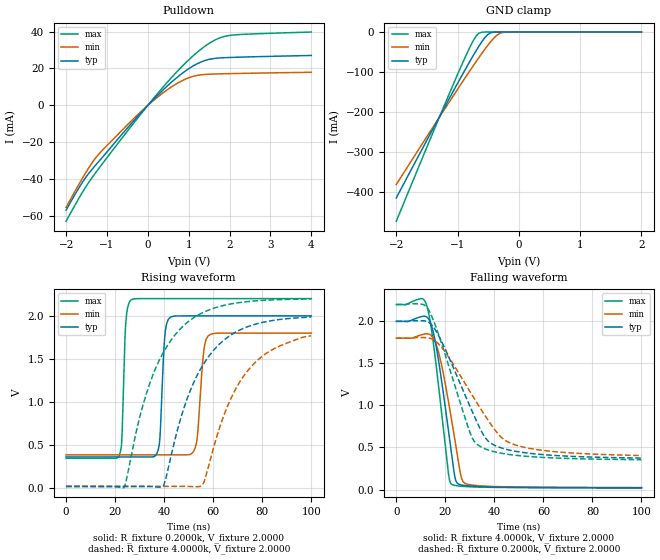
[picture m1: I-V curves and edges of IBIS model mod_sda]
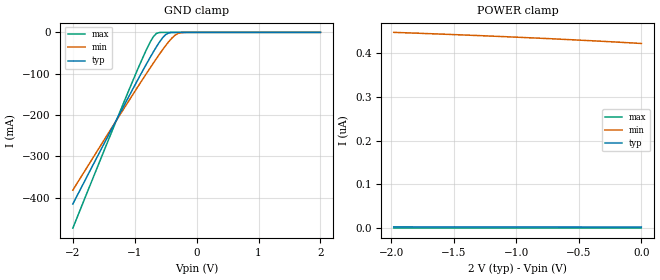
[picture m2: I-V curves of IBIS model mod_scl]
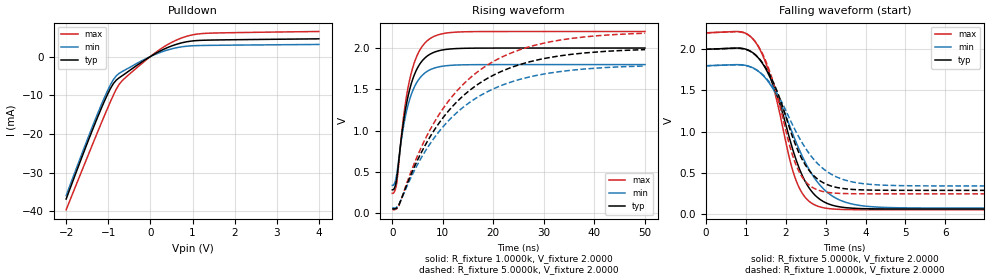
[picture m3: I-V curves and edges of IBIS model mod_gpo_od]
| IBIS (I/O, Buffer, Information, Specification) Model, officially
| electronic behavioral standard for Buffer structures of digital pins.
[IBIS ver]  4.0
[File name] st25dv04kc_so8_2v0.ibs
[File Rev]  1.0
[Date]   5 March 2024
[Notes]
   (Note1)  This IBIS model includes the SO8 package data
   (Note2)  This IBIS model has some Notes about the non-monotonicity
   of the I-V curves, but they are not indicative of problems
   inside the model;
[Disclaimer]
   Customers are solely responsible for all aspects of their
   own product designs or applications using this IBIS Model.
   STMicroelectronics assumes no liability for Custmer Designs
   and applications associated to this IBIS Model.
   In the use of this IBIS Model Customer shall not modify,
   disassemble, alter this Model in whole or in part.
   If Customers do not accept these terms, the IBIS Model
   may not be used. For any problems or modifications please
   contact STMicroelectronics (www.st.com).
[Copyright] (c) 2024 STMicroelectronics
|   Component ST25DV04K
[Component] ST25DV04K
[Manufacturer] STMicroelectronics
[Package]
| variable  typ   min   max
R_pkg   0.0   0.0   0.0
L_pkg   0.0H   0.0H   0.0H
C_pkg   0.0F   0.0F   0.0F
[Pin]  signal_name  model_name   R_pin   L_pin   C_pin
1   VEH   NC   0.0   0.0   0.0
2   AC0   NC   0.0   0.0   0.0
3   AC1   NC   0.0   0.0   0.0
4   VSS   GND   130.95m   2.182nH   0.287pF
5   SDA   mod_sda   130.79m   2.182nH   0.286pF
6   SCL   mod_scl   85.32m   1.589nH   0.354pF
7   GPO   mod_gpo_od   84.54m   1.583nH   0.355pF
8   VCC   POWER   124.14m   2.142nH   0.284pF
| Models and submodels in the file (3): mod_sda (I/O_open_drain), mod_scl (Input), mod_gpo_od (Open_drain)
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|   Model mod_sda
[Model]   mod_sda
Model_type I/O_open_drain
Polarity   Non-Inverting
Enable   Active-Low
Vinl   =   0.500V
Vinh   =   1.500V
Vmeas  =   1.000V
Cref   =   30.0pF
Rref   =   4.0k
Vref   =   2.000V
C_comp   3.063pF   2.925pF   3.207pF
[Model Spec]
Vmeas   1.000V   0.900V   1.100V
Vinl   0.500V   0.450V   0.550V
Vinh   1.500V   1.350V   1.650V
[Temperature Range]  25.0000   85.0000   -40.0000
[Voltage Range]   2.0000V   1.8000V   2.2000V
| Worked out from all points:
|   slope of the pulldown table from 0 to 0.3 V, typ, clamps not added: 44 ohm
|   GND clamp passes 1 mA (typ) near -0.44 V on its own axis
|   rising waveform, R_fixture 0.2000k, V_fixture 2.0000: 20-80 % time 1.54ns typ, 2.1ns min, 1.21ns max; typ from 0.364 V to 2 V
|   rising waveform, R_fixture 4.0000k, V_fixture 2.0000: 20-80 % time 16.8ns typ, 16.6ns min, 16.9ns max; typ from 0.021 V to 1.99 V
|   falling waveform, R_fixture 4.0000k, V_fixture 2.0000: 20-80 % time 5.73ns typ, 6.35ns min, 5.23ns max; typ from 2 V to 0.022 V
|   falling waveform, R_fixture 0.2000k, V_fixture 2.0000: 20-80 % time 14.7ns typ, 18.3ns min, 12.1ns max; typ from 2 V to 0.374 V
[Pulldown]
|Voltage   I(typ)   I(min)   I(max)
-2V       -56.79mA   -55.22mA   -62.78mA
-1.58V    -40.98mA   -38.72mA   -46.34mA
-1.3V     -32.95mA   -29.14mA   -37.16mA
-1.09V    -27.58mA   -23.79mA   -30.96mA
-390mV    -9.491mA   -8.101mA   -10.85mA
170mV     3.93mA     3.244mA    4.596mA
590mV     12.8mA     10.2mA     15.32mA
940mV     18.95mA    14.41mA    23.37mA
1.29V     23.41mA    16.53mA    30.26mA
1.64V     25.46mA    17.02mA    35.37mA
1.99V     25.95mA    17.21mA    37.85mA
4V        27.04mA    17.94mA    39.74mA
[GND_clamp]
|Voltage   I(typ)   I(min)   I(max)
-2V       -415.4mA   -381.8mA   -473.8mA
-1.35V    -227.6mA   -225.9mA   -232.7mA
-950mV    -114.5mA   -131.6mA   -88.58mA
-750mV    -60.32mA   -85.72mA   -23.2mA
-700mV    -47.4mA    -74.51mA   -10.46mA
-650mV    -34.97mA   -63.45mA   -2.549mA
-550mV    -13.06mA   -42.04mA   -27.64uA
-500mV    -5.297mA   -31.88mA   -2.458uA
-450mV    -1.324mA   -22.35mA   -217.9nA
-350mV    -35.28uA   -6.896mA   -1.714nA
-250mV    -802.3nA   -654.1uA   -15.76pA
2V        2.514nA    426.1nA    6.718pA
[Ramp]
| variable   typ   min   max
dV/dt_r   0.5972/2.3539n   0.4569/2.8918n   0.7297/1.3653n
dV/dt_f   0.5671/31.8553n   0.4108/32.1388n   0.7057/23.5150n
R_load = 50.0000
[Rising Waveform]
R_fixture= 0.2000k
V_fixture= 2.0000
V_fixture_min= 1.8000
V_fixture_max= 2.2000
|time   V(typ)   V(min)   V(max)
0s        363.6mV    387.8mV    348mV
21.66ns   363.6mV    387.8mV    378mV
24.4ns    363.6mV    387.8mV    1.937V
26.88ns   363.6mV    387.8mV    2.191V
37.52ns   440.7mV    387.8mV    2.2V
40.24ns   1.757V     387.8mV    2.2V
42.56ns   1.984V     387.8mV    2.2V
52.62ns   2V         466.6mV    2.2V
57.92ns   2V         1.768V     2.2V
100ns     2V         1.8V       2.2V
[Rising Waveform]
R_fixture= 4.0000k
V_fixture= 2.0000
V_fixture_min= 1.8000
V_fixture_max= 2.2000
|time   V(typ)   V(min)   V(max)
0s        21.01mV    22.65mV    19.91mV
23.68ns   21.01mV    22.65mV    8.087mV
31.38ns   21.01mV    22.65mV    967.1mV
39.22ns   15.66mV    22.65mV    1.552V
48.06ns   930.9mV    22.68mV    1.89V
55.46ns   1.415V     31.43mV    2.034V
65.36ns   1.741V     919.7mV    2.128V
73.16ns   1.865V     1.331V     2.163V
83.56ns   1.943V     1.599V     2.185V
100ns     1.986V     1.768V     2.196V
[Falling Waveform]
R_fixture= 4.0000k
V_fixture= 2.0000
V_fixture_min= 1.8000
V_fixture_max= 2.2000
|time   V(typ)   V(min)   V(max)
0s        2V         1.8V       2.2V
12.52ns   2.051V     1.852V     2.179V
14.8ns    1.905V     1.814V     1.811V
17.04ns   1.571V     1.653V     1.284V
21.3ns    696.3mV    1.042V     188.4mV
22.58ns   418.3mV    821.4mV    62.67mV
24.5ns    91.09mV    481.9mV    46.23mV
26.74ns   53.4mV     124.7mV    38.57mV
28.66ns   45.46mV    65.78mV    34.65mV
100ns     21.59mV    23.54mV    20.3mV
[Falling Waveform]
R_fixture= 0.2000k
V_fixture= 2.0000
V_fixture_min= 1.8000
V_fixture_max= 2.2000
|time   V(typ)   V(min)   V(max)
0s        2V         1.8V       2.2V
9.72ns    2.008V     1.807V     2.208V
12.78ns   1.995V     1.804V     2.154V
18.68ns   1.749V     1.683V     1.718V
30.24ns   977.1mV    1.156V     664.1mV
34.44ns   708.7mV    958.8mV    508.4mV
37.24ns   581.8mV    833.1mV    472.7mV
42.84ns   494.9mV    620.4mV    431.7mV
49.84ns   448.8mV    519.2mV    403.7mV
100ns     374.2mV    404.2mV    354.8mV
|   Model mod_scl
[Model]   mod_scl
Model_type Input
Vinl   =   0.500V
Vinh   =   1.500V
C_comp   2.118pF   2.024pF   2.219pF
[Model Spec]
Vinl   0.500V   0.450V   0.550V
Vinh   1.500V   1.350V   1.650V
[Temperature Range]  25.0000   85.0000   -40.0000
[Voltage Range]   2.0000V   1.8000V   2.2000V
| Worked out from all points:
|   GND clamp passes 1 mA (typ) near -0.44 V on its own axis
[GND_clamp]
|Voltage   I(typ)   I(min)   I(max)
-2V       -415.4mA   -381.8mA   -473.8mA
-1.35V    -227.6mA   -225.9mA   -232.7mA
-950mV    -114.5mA   -131.6mA   -88.58mA
-750mV    -60.32mA   -85.72mA   -23.2mA
-700mV    -47.4mA    -74.51mA   -10.46mA
-650mV    -34.97mA   -63.45mA   -2.549mA
-550mV    -13.06mA   -42.04mA   -27.64uA
-500mV    -5.297mA   -31.88mA   -2.458uA
-450mV    -1.324mA   -22.35mA   -217.9nA
-350mV    -35.28uA   -6.896mA   -1.714nA
-250mV    -802.3nA   -654.1uA   -15.76pA
2V        2.514nA    426.1nA    6.718pA
[POWER_clamp]
|Voltage   I(typ)   I(min)   I(max)
-1.98V    2.873nA    448.3nA    11.48pA
-1.77V    2.841nA    446.2nA    11.03pA
-1.38V    2.78nA     441.9nA    10.19pA
-1.11V    2.734nA    438.7nA    9.602pA
-870mV    2.691nA    435.6nA    9.079pA
-840mV    2.686nA    435.3nA    9.014pA
-690mV    2.658nA    433.3nA    8.685pA
-360mV    2.592nA    428.6nA    7.961pA
0V        2.514nA    422.9nA    7.164pA
|   Model mod_gpo_od
[Model]   mod_gpo_od
Model_type Open_drain
Polarity   Non-Inverting
Enable   Active-Low
Vmeas  =   1.000V
Cref   =   30.0pF
Rref   =   5.0k
Vref   =   2.00V
C_comp   2.219pF   2.119pF   2.324pF
[Model Spec]
Vmeas   1.000V   0.900V   1.100V
[Temperature Range]  25.0000   85.0000   -40.0000
[Voltage Range]   2.0000V   1.8000V   2.2000V
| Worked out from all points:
|   slope of the pulldown table from 0 to 0.3 V, typ, clamps not added: 168 ohm
|   rising waveform, R_fixture 1.0000k, V_fixture 2.0000: 20-80 % time 2.97ns typ, 2.98ns min, 2.96ns max; typ from 0.286 V to 2 V
|   rising waveform, R_fixture 5.0000k, V_fixture 2.0000: 20-80 % time 14.3ns typ, 14.3ns min, 14.3ns max; typ from 0.059 V to 1.98 V
|   falling waveform, R_fixture 5.0000k, V_fixture 2.0000: 20-80 % time 784ps typ, 989ps min, 658ps max; typ from 2 V to 0.059 V
|   falling waveform, R_fixture 1.0000k, V_fixture 2.0000: 20-80 % time 817ps typ, 1.03ns min, 686ps max; typ from 2 V to 0.286 V
[Pulldown]
|Voltage   I(typ)   I(min)   I(max)
-2V       -36.84mA   -35.95mA   -39.62mA
-1.58V    -24.7mA    -23.82mA   -28.25mA
-1.3V     -16.94mA   -16.03mA   -20.76mA
-1.02V    -9.839mA   -8.885mA   -13.45mA
-880mV    -7.009mA   -5.99mA    -10.01mA
-740mV    -5.488mA   -4.339mA   -7.151mA
-670mV    -4.961mA   -3.875mA   -6.241mA
170mV     1.07mA     795.9uA    1.404mA
660mV     3.293mA    2.356mA    4.451mA
870mV     3.825mA    2.675mA    5.258mA
1.15V     4.157mA    2.837mA    5.853mA
4V        4.574mA    3.119mA    6.471mA
[Ramp]
| variable   typ   min   max
dV/dt_r   0.1294/0.8382n   87.4200m/0.8549n   0.1846/0.8357n
dV/dt_f   0.1297/0.7724n   87.6000m/0.7721n   0.1844/0.7711n
R_load = 50.0000
[Rising Waveform]
R_fixture= 1.0000k
V_fixture= 2.0000
V_fixture_min= 1.8000
V_fixture_max= 2.2000
|time   V(typ)   V(min)   V(max)
0s        285.8mV    339.1mV    243.3mV
500ps     318.4mV    372.2mV    273.6mV
900ps     428.5mV    481.6mV    375.9mV
2.3ns     1.143V     1.081V     1.201V
3ns       1.384V     1.283V     1.483V
3.7ns     1.558V     1.429V     1.685V
5.3ns     1.793V     1.626V     1.959V
7.5ns     1.927V     1.738V     2.115V
13.9ns    1.996V     1.797V     2.196V
50ns      2V         1.8V       2.2V
[Rising Waveform]
R_fixture= 5.0000k
V_fixture= 2.0000
V_fixture_min= 1.8000
V_fixture_max= 2.2000
|time   V(typ)   V(min)   V(max)
0s        59.08mV    70.65mV    49.99mV
1.3ns     100.9mV    108.4mV    93.46mV
5.1ns     658.7mV    603.5mV    714mV
9.1ns     1.08V      978.9mV    1.182V
13.1ns    1.37V      1.237V     1.503V
17.7ns    1.592V     1.435V     1.749V
23.15ns   1.757V     1.582V     1.931V
30.3ns    1.876V     1.689V     2.064V
38.25ns   1.942V     1.748V     2.136V
50ns      1.981V     1.783V     2.179V
[Falling Waveform]
R_fixture= 5.0000k
V_fixture= 2.0000
V_fixture_min= 1.8000
V_fixture_max= 2.2000
|time   V(typ)   V(min)   V(max)
0s        2V         1.8V       2.2V
900ps     2.012V     1.812V     2.211V
1.26ns    1.924V     1.753V     2.076V
1.66ns    1.602V     1.539V     1.599V
2.26ns    658.8mV    873mV      407.5mV
2.5ns     384.7mV    617.4mV    194.8mV
2.86ns    175.5mV    348.4mV    84.31mV
3.46ns    77.84mV    147.9mV    52.94mV
4.38ns    60.16mV    80.29mV    50.05mV
15ns      59.07mV    70.65mV    49.99mV
[Falling Waveform]
R_fixture= 1.0000k
V_fixture= 2.0000
V_fixture_min= 1.8000
V_fixture_max= 2.2000
|time   V(typ)   V(min)   V(max)
0s        2V         1.8V       2.2V
880ps     2.011V     1.81V      2.21V
1.24ns    1.933V     1.758V     2.092V
1.64ns    1.652V     1.572V     1.677V
2.28ns    800.6mV    978.9mV    571.1mV
2.52ns    574.2mV    781.1mV    381.6mV
2.88ns    395.4mV    574.1mV    278.2mV
3.52ns    303.3mV    406mV      246.1mV
4.48ns    286.8mV    348.2mV    243.3mV
15ns      285.8mV    339.1mV    243.3mV
